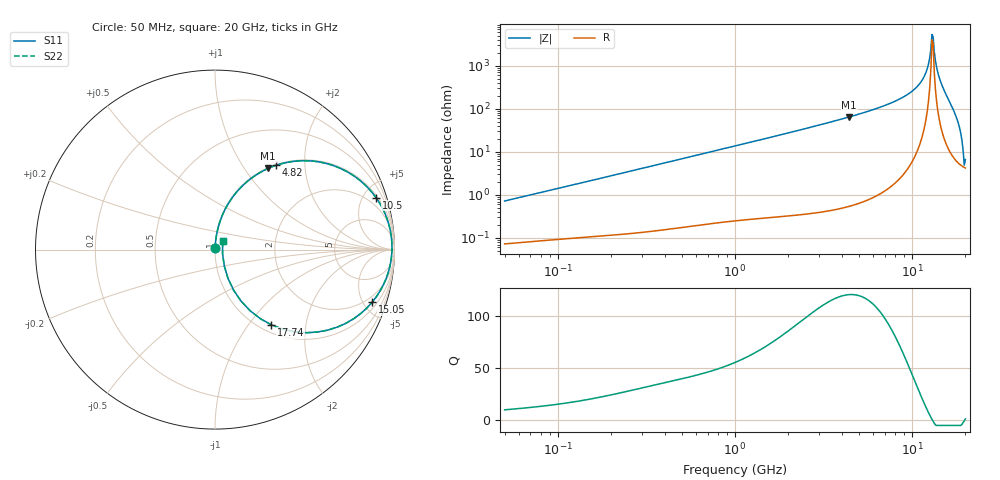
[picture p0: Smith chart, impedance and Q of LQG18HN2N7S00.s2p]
!Murata Part Number: LQG18HN2N7S00
!These Parameters are Measured in Series Mode Connection
!  o--[Z]--o
!Port1  Port2
!  o-------o
!Freq. Start=50[MHz] Stop=20[GHz], 401[Steps]
# Hz S RI R 50
!Freq.(Hz) S11(Real) S11(Imag) S21(Real) S21(Imag) S12(Real) S12(Imag) S22(Real) S22(Imag)
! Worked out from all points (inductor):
!   401 points, 50 MHz to 20 GHz, reference 50 ohm
!   read as one part in series: L = 2.26 nH near 51.52 MHz
!   highest Q = 120 at 4.406 GHz (marker M1), where L = 2.33 nH
!   self-resonance near 12.95 GHz
!   S11 on the Smith chart (normalised r, x): 50 MHz: 1.00, +0.01; 4.82 GHz: 1.01, +1.44; 10.5 GHz: 1.18, +6.13; 15.05 GHz: 1.45, -5.78; 17.74 GHz: 1.12, -1.30; 20 GHz: 1.08, +0.10
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5e7  0.000773 0.00715  0.9992 -0.00715  0.9992 -0.00715  0.000773 0.00715
1.364002e8  0.00138 0.019  0.9986 -0.019  0.9986 -0.019  0.00138 0.019
3.721004e8  0.0041 0.051  0.9959 -0.051  0.9959 -0.051  0.0041 0.051
1e9  0.0207 0.1337  0.9793 -0.1337  0.9793 -0.1337  0.0207 0.1337
2.728004e9  0.129 0.3304  0.871 -0.3304  0.871 -0.3304  0.129 0.3304
4.405649e9  0.2961 0.4524  0.7039 -0.4524  0.7039 -0.4524  0.2961 0.4524
4.81993e9  0.3421 0.4703  0.6579 -0.4703  0.6579 -0.4703  0.3421 0.4703
7.442007e9  0.633 0.4765  0.367 -0.4765  0.367 -0.4765  0.633 0.4765
1.050288e10  0.8971 0.2899  0.1029 -0.2899  0.1029 -0.2899  0.8971 0.2899
1.183995e10  0.9649 0.1522  0.0351 -0.1522  0.0351 -0.1522  0.9649 0.1522
1.220001e10  0.9759 0.1093  0.0241 -0.1093  0.0241 -0.1093  0.9759 0.1093
1.276073e10  0.9853 0.0378  0.0147 -0.0378  0.0147 -0.0378  0.9853 0.0378
1.295331e10  0.986 0.012  0.014 -0.012  0.014 -0.012  0.986 0.012
1.334722e10  0.9829 -0.0428  0.0171 0.0428  0.0171 0.0428  0.9829 -0.0428
1.375312e10  0.9725 -0.1015  0.0275 0.1015  0.0275 0.1015  0.9725 -0.1015
1.417136e10  0.9527 -0.1636  0.0473 0.1636  0.0473 0.1636  0.9527 -0.1636
1.504638e10  0.8756 -0.2933  0.1244 0.2933  0.1244 0.2933  0.8756 -0.2933
1.646126e10  0.6286 -0.4486  0.3714 0.4486  0.3714 0.4486  0.6286 -0.4486
1.774144e10  0.3145 -0.4193  0.6855 0.4193  0.6855 0.4193  0.3145 -0.4193
1.855685e10  0.1453 -0.287  0.8547 0.287  0.8547 0.287  0.1453 -0.287
1.940974e10  0.0518 -0.0914  0.9482 0.0914  0.9482 0.0914  0.0518 -0.0914
2e10  0.0426 0.0472  0.9574 -0.0472  0.9574 -0.0472  0.0426 0.0472
